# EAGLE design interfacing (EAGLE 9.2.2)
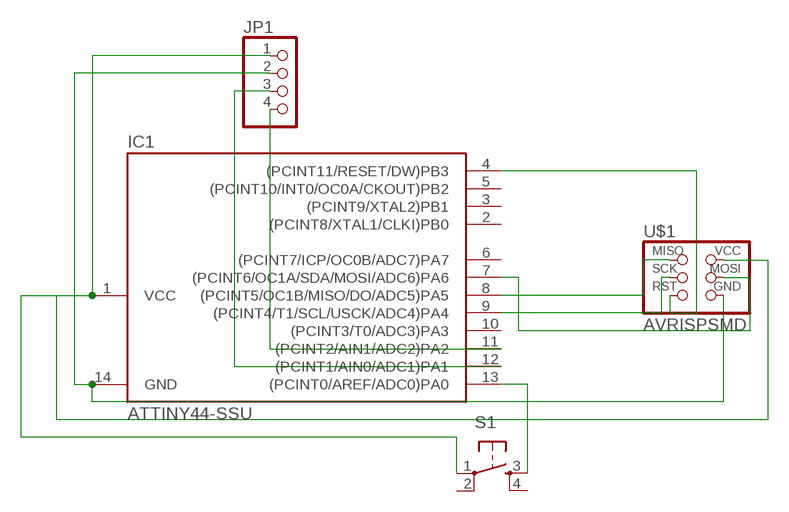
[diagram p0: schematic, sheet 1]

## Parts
IC1  ATTINY44-SSU  [SOIC14]
JP1  PINHD-1X4  [1X04]
S1  6MM_SWITCH6MM_SWITCH  [6MM_SWITCH]
U$1  AVRISPSMD  [2X03SMD]

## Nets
N$1: IC1.8((PCINT5/OC1B/MISO/DO/ADC5)PA5) U$1.1(MISO)
N$2: IC1.9((PCINT4/T1/SCL/USCK/ADC4)PA4) U$1.3(SCK)
N$3: IC1.4((PCINT11/RESET/DW)PB3) U$1.5(RST)
N$4: IC1.7((PCINT6/OC1A/SDA/MOSI/ADC6)PA6) U$1.4(MOSI)
N$5: IC1.1(VCC) JP1.1 S1.1(P) U$1.2(VCC)
N$6: IC1.14(GND) JP1.2 U$1.6(GND)
N$7: IC1.13((PCINT0/AREF/ADC0)PA0) S1.3(S)
N$8: IC1.12((PCINT1/AIN0/ADC1)PA1) JP1.3
N$9: IC1.11((PCINT2/AIN1/ADC2)PA2) JP1.4
Unconnected: IC1.2((PCINT8/XTAL1/CLKI)PB0) IC1.3((PCINT9/XTAL2)PB1) IC1.5((PCINT10/INT0/OC0A/CKOUT)PB2) IC1.6((PCINT7/ICP/OC0B/ADC7)PA7) IC1.10((PCINT3/T0/ADC3)PA3) S1.2(P1) S1.4(S1)

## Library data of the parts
IC1 = fab:ATTINY44
JP1 = pinhead:PINHD-1X4: PIN HEADER
S1 = fab:6MM_SWITCH: OMRON SWITCH
U$1 = fab:AVRISP

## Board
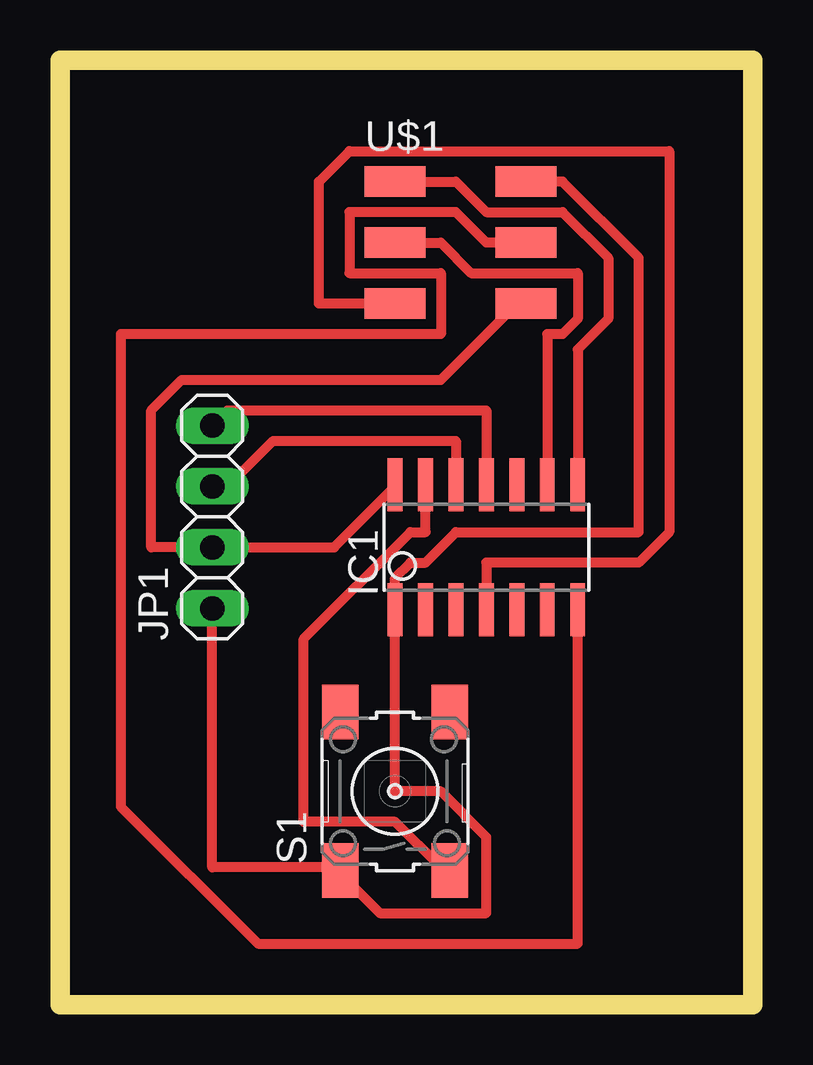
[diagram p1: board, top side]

Size 28.88 x 39.36 mm. Coordinates in mm from the lower left corner, seen from the top.
Outline: 0,0 28.88,0 28.88,39.36 0,39.36 0,0
Copper layers (1*16): Top 0.035mm / dielectric 1.5mm / Bottom 0.035mm
Design rules "default *": minimum track width 16mil, minimum drill 0.35mm, track to track 16mil, track to pad 16mil, pad to pad 16mil, via to via 16mil, smd to smd 16mil, copper to edge 40mil, drill to drill 16mil, minimum pad ring 10mil, minimum via ring 8mil, stop-mask expansion 4mil, vias tented up to drill 0mil, thermal gap 10mil

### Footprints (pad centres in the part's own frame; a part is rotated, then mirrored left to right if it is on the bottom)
SOIC14 = smd 0.61 x 2.21: 1 -3.81,-2.603; 2 -2.54,-2.603; 3 -1.27,-2.603; 4 0,-2.603; 5 1.27,-2.603; 6 2.54,-2.603; 7 3.81,-2.603; 8 3.81,2.603; 9 2.54,2.603; 10 1.27,2.603; 11 0,2.603; 12 -1.27,2.603; 13 -2.54,2.603; 14 -3.81,2.603
1X04 = drill 1.016 long: 1 -3.81,0; 2 -1.27,0; 3 1.27,0; 4 3.81,0
6MM_SWITCH = smd 2.286 x 1.524: 1 -3.302,2.286; 2 3.302,2.286; 3 -3.302,-2.286; 4 3.302,-2.286
2X03SMD = smd 2.54 x 1.27: 1 -2.54,2.54; 2 2.92,2.54; 3 -2.54,0; 4 2.92,0; 5 -2.54,-2.54; 6 2.92,-2.54

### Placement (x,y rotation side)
IC1  17.78,19.05 0 top
JP1  6.35,20.32 90 top
S1  13.97,8.89 90 top
U$1  16.51,31.75 0 top

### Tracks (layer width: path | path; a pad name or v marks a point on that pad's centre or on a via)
N$1
  Top 0.406: IC1.8 21.59,27.3 22.86,28.57 22.86,31.11 20.95,33.02 17.78,33.02 16.51,34.29 U$1.1
N$2
  Top 0.406: IC1.9 20.32,27.94 20.95,27.94 21.59,28.57 21.59,30.48 17.15,30.48 15.88,31.75 U$1.3
N$3
  Top 0.406: IC1.4 17.78,18.41 24.13,18.41 25.4,19.68 25.4,35.56 12.06,35.56 10.8,34.29 10.8,29.21 U$1.5
N$4
  Top 0.406: IC1.7 21.59,2.54 8.26,2.54 2.54,8.25 2.54,27.94 15.88,27.94 15.88,30.48 12.06,30.48 12.06,33.02 16.51,33.02 17.78,31.75 U$1.4
N$5
  Top 0.406: U$1.2 20.95,34.29 24.13,31.11 24.13,19.68 16.51,19.68 15.24,18.41 14.61,18.41 13.97,17.78 IC1.1 13.97,8.89 15.88,8.89 17.78,6.98 17.78,3.81 13.34,3.81 12.06,5.08 S1.1 11.43,5.71 6.35,5.71 JP1.1
N$6
  Top 0.406: IC1.14 13.97,21.59 11.43,19.05 JP1.2 3.81,19.05 3.81,24.76 5.08,26.04 15.88,26.04 19.05,29.21 U$1.6
N$7
  Top 0.406: IC1.13 15.24,19.68 14.61,19.68 10.16,15.24 10.16,7.62 13.97,7.62 15.88,5.71 S1.3
N$8
  Top 0.406: IC1.12 16.51,23.5 8.89,23.5 6.98,21.59 JP1.3
N$9
  Top 0.406: IC1.11 17.78,24.76 6.98,24.76 JP1.4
